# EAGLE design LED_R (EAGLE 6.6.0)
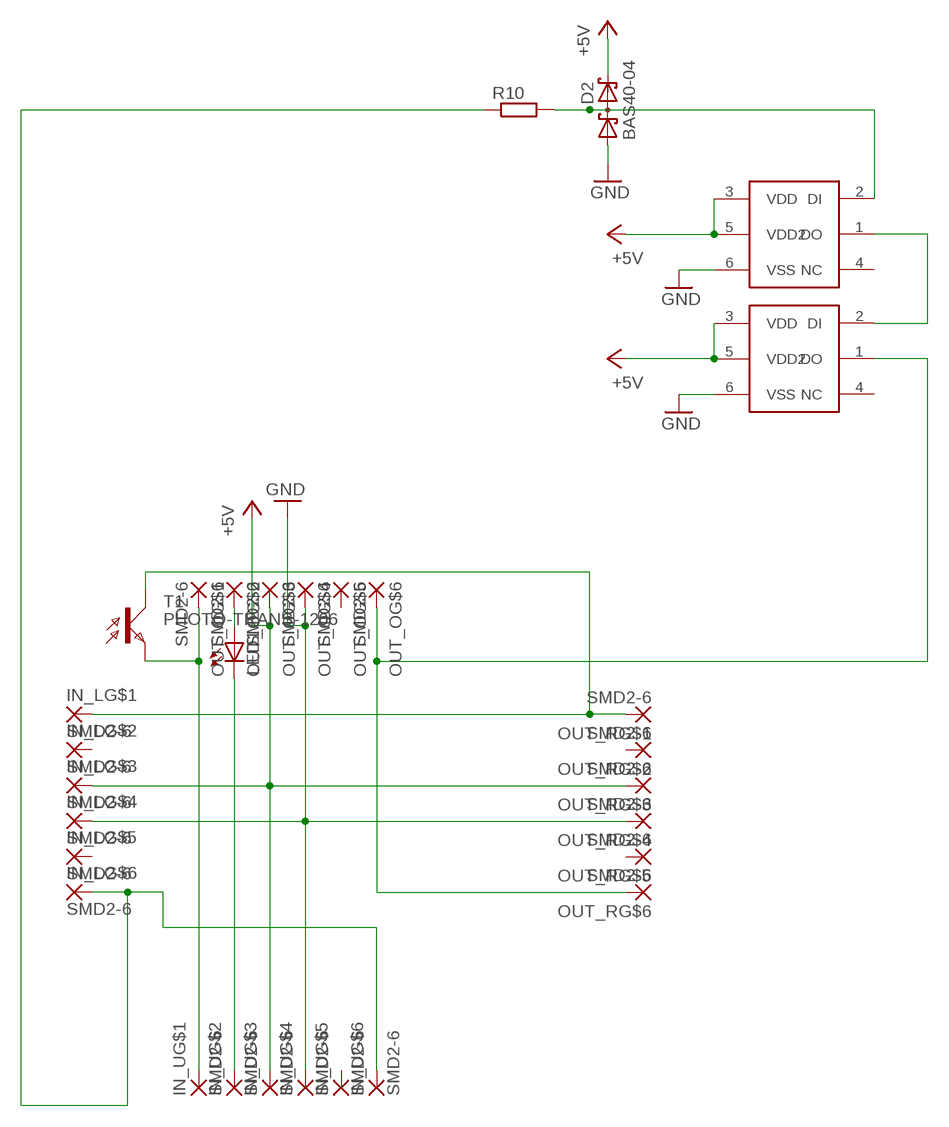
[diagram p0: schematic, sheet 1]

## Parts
D2  BAS40-04  [SOT23]
IN_L  SMD2-6  [SMD1,27-2,54-6]
IN_U  SMD2-6  [SMD1,27-2,54-6]
LED1  LED3MM  [LED3MM]
OUT_O  SMD2-6  [SMD1,27-2,54-6]
OUT_R  SMD2-6  [SMD1,27-2,54-6]
R10  R-EU_M1206  [M1206]
T1  PHOTO-TRANS-1206  [1206]
U$1  LED_SMD5050  [CLN6A]
U$2  LED_SMD5050  [CLN6A]

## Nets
+5V: D2.2(C2) IN_L.3 IN_U.3 OUT_O.3 OUT_R.3 U$1.3(VDD) U$1.5(VDD2) U$2.3(VDD) U$2.5(VDD2)
GND: D2.1(A1) IN_L.4 IN_U.4 OUT_O.4 OUT_R.4 U$1.6(VSS) U$2.6(VSS)
N$4: IN_U.1 OUT_O.1 T1.C(E)
N$6: U$1.1(DO) U$2.2(DI)
N$7: D2.3(C1A2) R10.2 U$1.2(DI)
N$13: LED1.A OUT_O.2
N$17: IN_L.6 IN_U.6 R10.1
N$18: IN_L.1 OUT_R.1 T1.A(C)
N$21: OUT_O.6 OUT_R.6 U$2.1(DO)
N$25: IN_U.2 LED1.K(C)
Unconnected: IN_L.2 IN_L.5 IN_U.5 OUT_O.5 OUT_R.2 OUT_R.5 U$1.4(NC) U$2.4(NC)

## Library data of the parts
D2 = diode:BAS40-04: Silicon Schottky Diodes General-purpose diode for high-speed switching
IN_L IN_U OUT_O OUT_R = #mylib:SMD2-6
LED1 = led:LED: LED
R10 = resistor:R-EU_: RESISTOR, European symbol
T1 = #mylib:PHOTO-TRANS-1206: PHOTO TRANSISTOR
U$1 U$2 = #mylib:LED_SMD5050

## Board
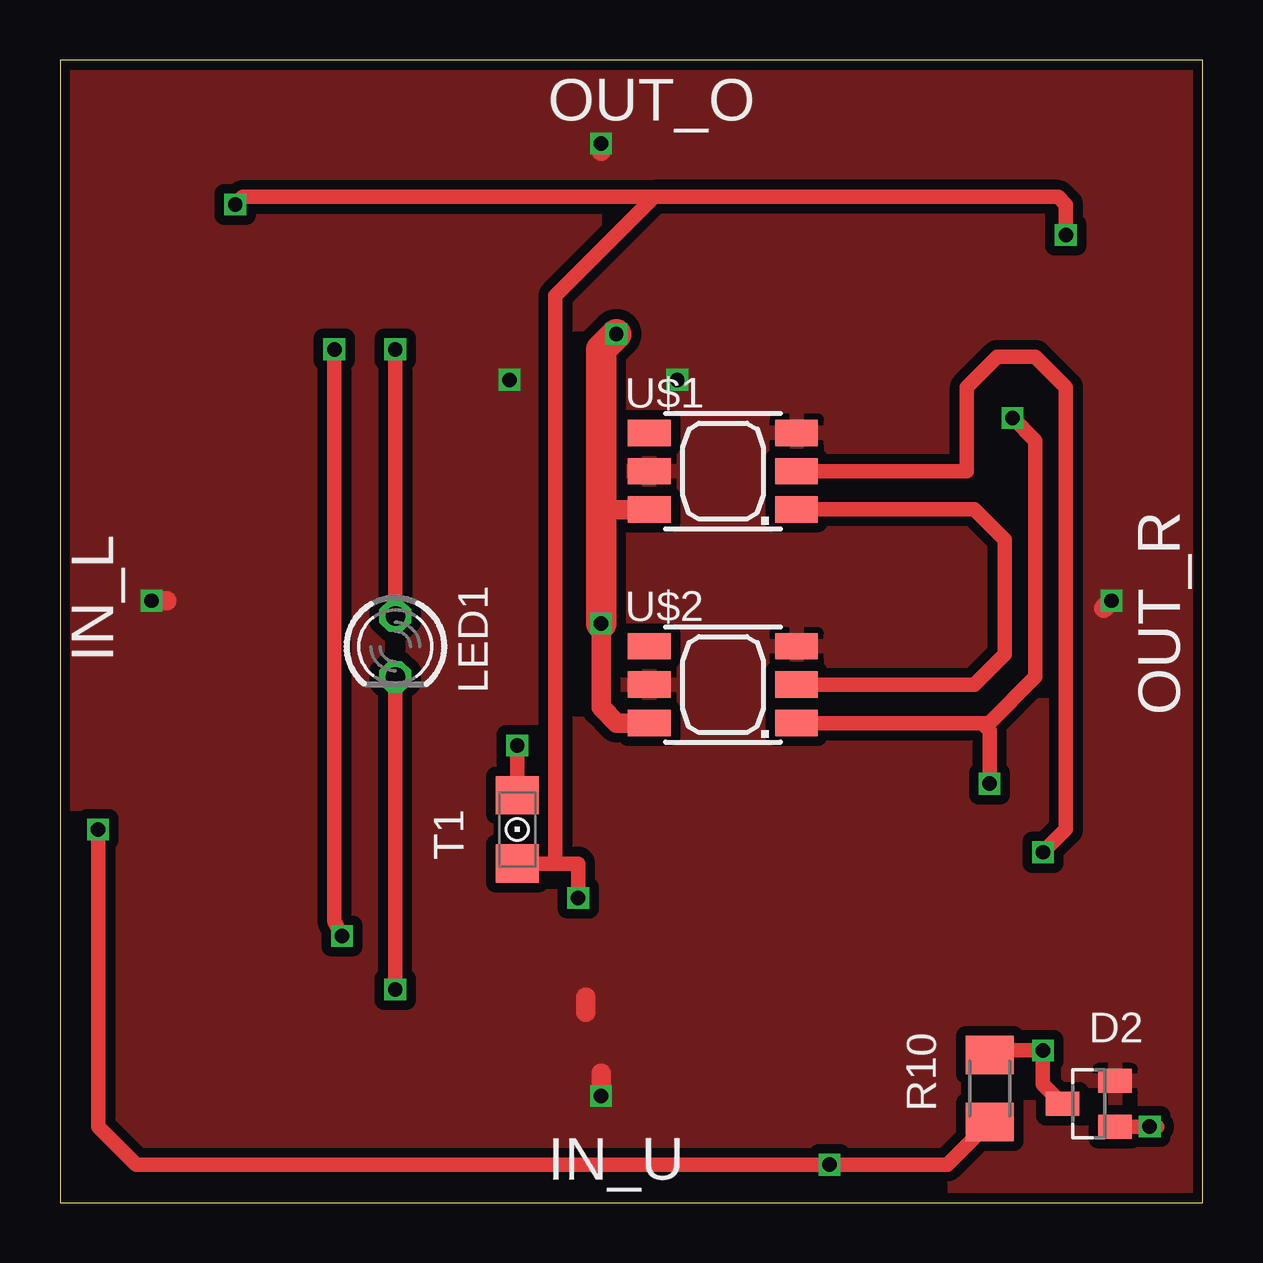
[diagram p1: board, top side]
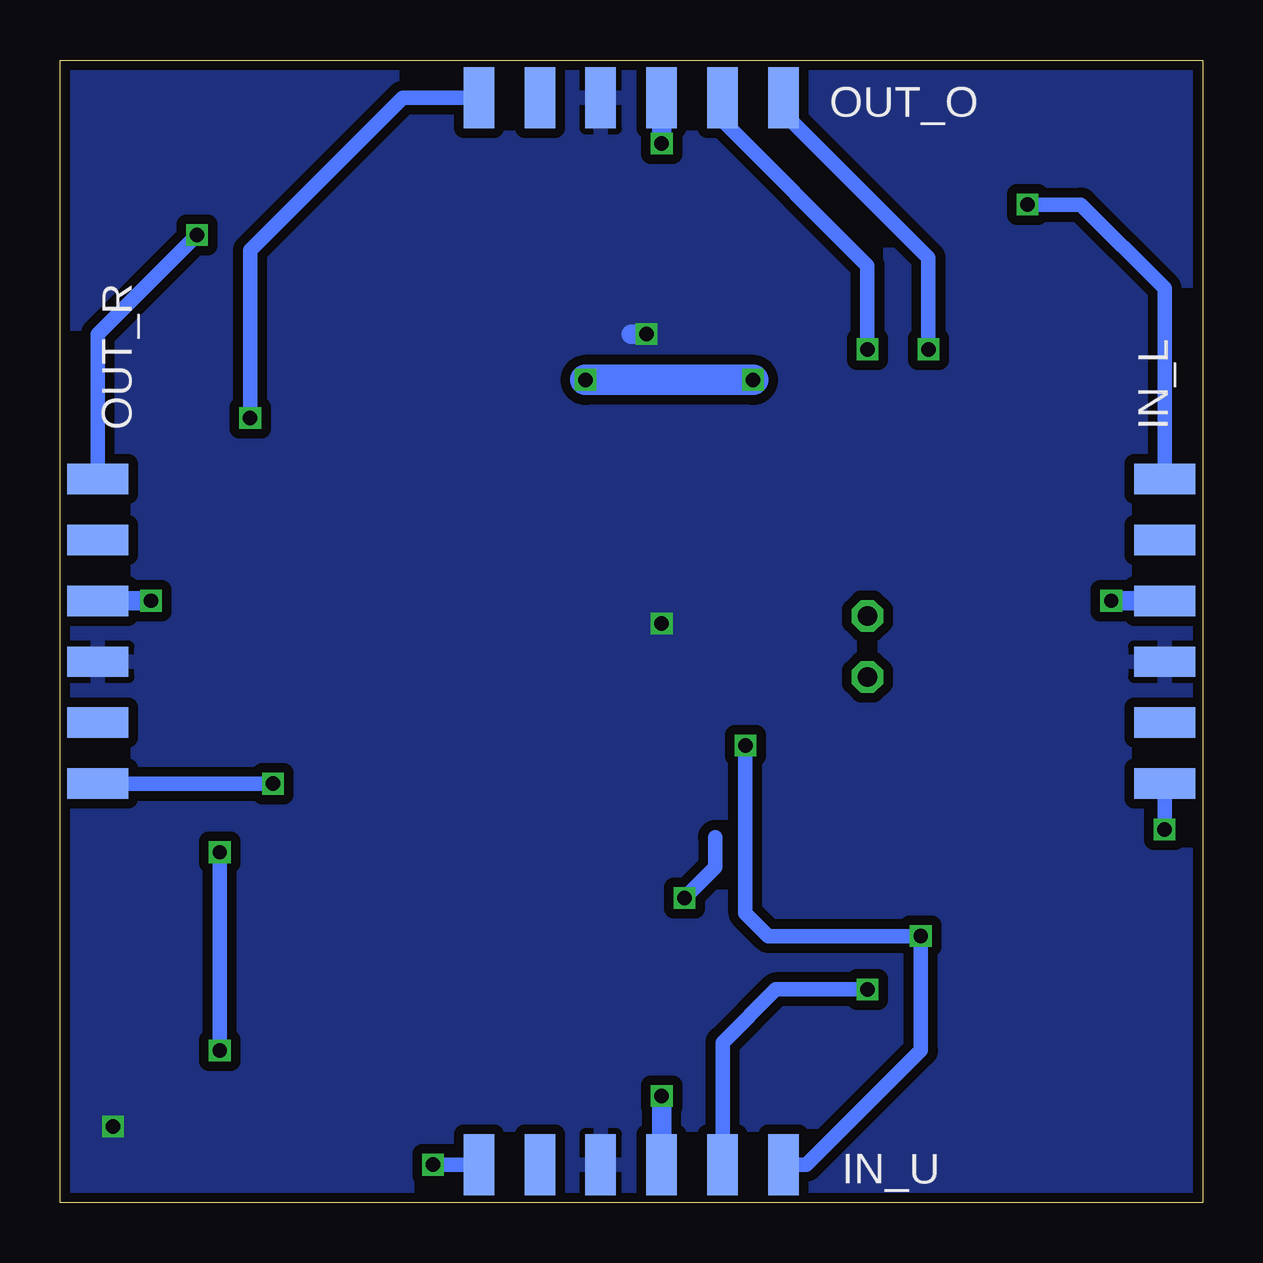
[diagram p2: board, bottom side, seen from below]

Size 47.61 x 47.62 mm. Coordinates in mm from the lower left corner, seen from the top.
Outline: 0,0 47.61,0 47.61,47.62 0,47.62 0,0
Copper layers (1*16): Top 0.035mm / dielectric 1.5mm / Bottom 0.035mm
Design rules "Elecrow_2-layer_eagle_rule": minimum track width 6mil, minimum drill 12mil, track to track 6mil, track to pad 6mil, pad to pad 6mil, via to via 6mil, smd to smd 0mil, copper to edge 10mil, drill to drill 10mil, minimum pad ring 10mil, minimum via ring 6mil, stop-mask expansion 2mil, vias tented up to drill 100mil, thermal gap 10mil

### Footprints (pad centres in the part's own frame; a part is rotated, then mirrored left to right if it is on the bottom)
SOT23 = smd 1 x 1.4: 1 -0.95,-1.1; 2 0.95,-1.1; 3 0,1.1
SMD1,27-2,54-6 = smd 1.27 x 2.54: 1 0,0; 2 2.54,0; 3 5.08,0; 4 7.62,0; 5 10.16,0; 6 12.7,0
LED3MM = drill 0.813 octagon: A -1.27,0; K 1.27,0
M1206 = smd 1.6 x 2: 1 -1.4,0; 2 1.4,0
1206 = smd 1.6 x 1.803: A -1.422,0; C 1.422,0
CLN6A = smd 1.778 x 1.1: 1 3.071,-1.6; 2 3.071,0; 3 3.071,1.6; 4 -3.071,1.6; 5 -3.071,0; 6 -3.071,-1.6

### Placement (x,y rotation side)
D2  42.86,4.13 90 top
IN_L  1.59,30.16 270 bottom
IN_U  17.46,1.59 180 bottom
LED1  13.97,23.18 270 top
OUT_O  17.46,46.04 180 bottom
OUT_R  46.04,30.16 270 bottom
R10  38.73,4.76 90 top
T1  19.05,15.56 90 top
U$1  27.62,30.48 0 top
U$2  27.62,21.59 0 top

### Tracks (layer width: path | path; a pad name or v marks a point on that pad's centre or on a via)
+5V  (via drill 0.6)
  Top 0.813: 21.91,7.94 21.91,8.57 | v43.81,25.08 43.5,24.77 | v22.54,4.45 22.54,5.4 | v3.81,25.08 4.45,25.08 | v22.54,44.13 22.54,43.81
  Bottom 0.813: OUT_R.3 v43.81,25.08 | IN_U.3 v22.54,4.45 | IN_L.3 v3.81,25.08 | OUT_O.3 v22.54,44.13
  Bottom 1.27: v18.73,34.29 v25.72,34.29
  pour Top (isolate 0.406): 0.32,47.31 47.31,47.31 47.31,0.32 0.32,0.32
GND  (via drill 0.6)
  Top 0.61: D2.1 45.72,3.18 v45.4,3.17
  Top 0.813: U$2.6 23.19,19.99 22.54,20.64 v22.54,24.13 | U$1.6 22.55,28.88 22.54,28.89
  Top 1.27: v22.54,24.13 22.54,28.89 22.54,35.56 v23.18,36.2
  Bottom 0.813: v23.18,36.2 23.81,36.2
  pour Bottom (isolate 0.406): 0.32,47.31 47.31,47.31 47.31,0.32 0.32,0.32
N$4  (via drill 0.6)
  Top 0.61: v11.43,35.56 11.43,11.75 v11.75,11.11 | v19.05,19.05 T1.C
  Bottom 0.61: v11.43,35.56 11.43,39.37 13.02,40.96 13.34,41.27 17.46,45.4 OUT_O.1 | v19.05,19.05 19.05,12.06 18.1,11.11 v11.75,11.11 11.75,6.35 16.51,1.59 IN_U.1
N$6
  Top 0.61: U$2.2 38.1,21.59 39.37,22.86 39.37,27.62 38.1,28.89 30.71,28.89 U$1.1
N$7  (via drill 0.6)
  Top 0.61: 41.91,3.98 D2.3 40.96,4.93 v40.96,6.35 38.92,6.35 R10.2 | U$1.2 37.78,30.48 37.78,33.97 39.05,35.24 40.64,35.24 41.91,33.97 41.91,15.56 v40.96,14.61
  Bottom 0.61: v40.96,6.35 v40.96,14.61
N$13  (via drill 0.6)
  Top 0.61: v13.97,35.56 LED1.A
  Bottom 0.61: v13.97,35.56 13.97,39.05 20,45.09 OUT_O.2
N$17  (via drill 0.6)
  Top 0.61: R10.1 36.96,1.59 v32.07,1.59 3.17,1.59 1.59,3.17 v1.59,15.56
  Bottom 0.61: IN_U.6 v32.07,1.59 | IN_L.6 v1.59,15.56
N$18  (via drill 0.6)
  Top 0.61: v21.59,12.7 21.59,14.14 T1.A 20.64,14.14 20.64,37.78 24.77,41.91 | v41.91,40.32 41.91,41.59 41.59,41.91 24.77,41.91 | v7.3,41.59 7.62,41.91 24.77,41.91
  Bottom 0.61: 20.32,15.24 20.32,13.97 v21.59,12.7 | OUT_R.1 46.04,36.2 v41.91,40.32 | v7.3,41.59 5.08,41.59 1.59,38.1 IN_L.1
N$21  (via drill 0.6)
  Top 0.61: U$2.1 38.42,19.99 | 38.42,19.99 38.72,19.99 40.64,21.91 40.64,31.75 v39.69,32.7 | v38.73,17.46 38.73,19.67 38.42,19.99
  Bottom 0.61: v39.69,32.7 39.69,39.69 33.34,46.04 OUT_O.6 | OUT_R.6 v38.73,17.46
N$25  (via drill 0.6)
  Top 0.61: v13.97,8.89 LED1.K
  Bottom 0.61: v13.97,8.89 17.78,8.89 20,6.67 IN_U.2

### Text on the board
tNames: OUT_O | IN_L | OUT_R | IN_U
